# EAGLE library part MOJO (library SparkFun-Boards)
Mojo v3 FPGA Development Board Mechanical footprint with connectors for Mojo FPGA dev board. SparkFun Products: Mojo v3
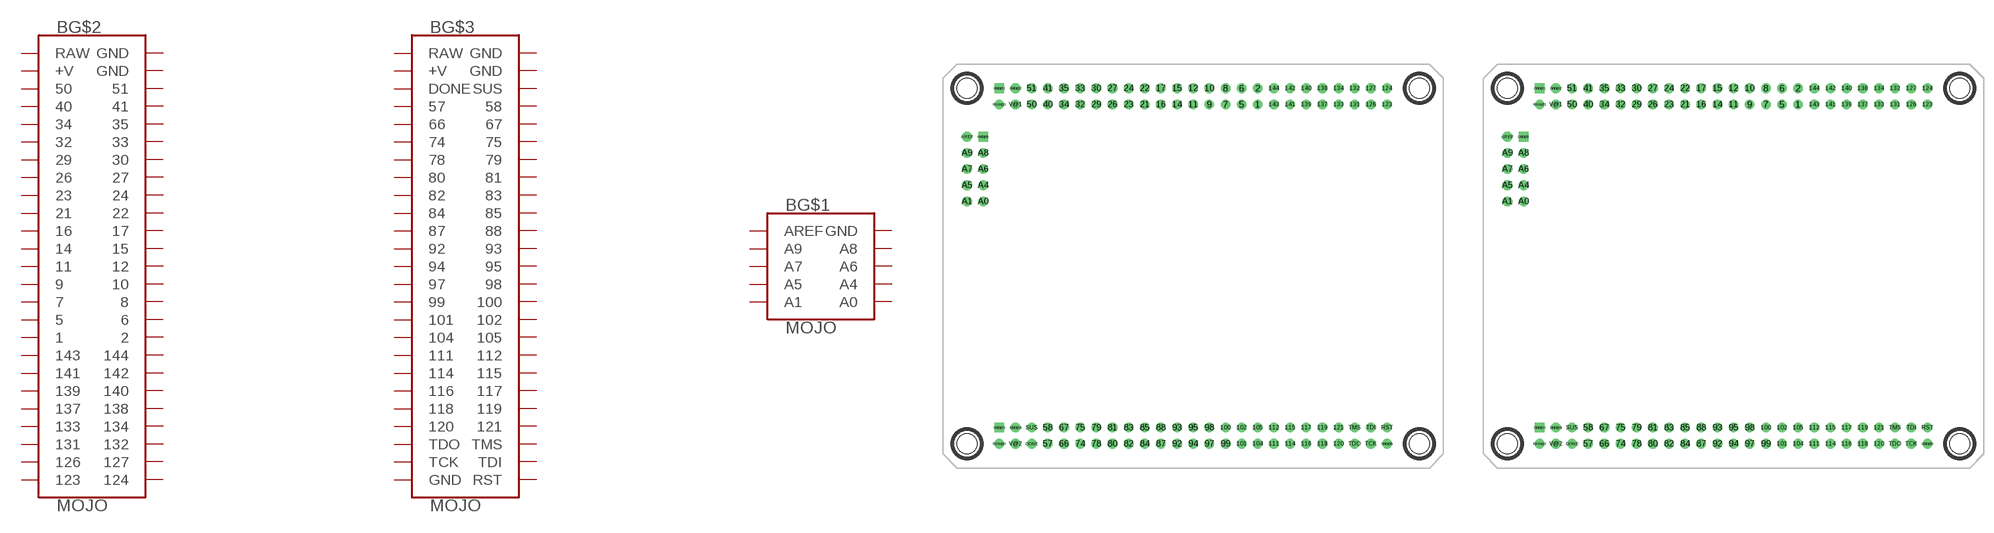
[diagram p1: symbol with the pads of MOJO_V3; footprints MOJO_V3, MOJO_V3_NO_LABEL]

Designator prefix B; gates G$1=MOJO_ANALOG_HEADER G$2=MOJO_HEADER_1 G$3=MOJO_HEADER_2

## MOJOV3  [MOJO_V3]
1  G$2:1
2  G$2:2
5  G$2:5
6  G$2:6
7  G$2:7
8  G$2:8
9  G$2:9
10  G$2:10
11  G$2:11
12  G$2:12
14  G$2:14
15  G$2:15
16  G$2:16
17  G$2:17
21  G$2:21
22  G$2:22
23  G$2:23
24  G$2:24
26  G$2:26
27  G$2:27
29  G$2:29
30  G$2:30
32  G$2:32
33  G$2:33
34  G$2:34
35  G$2:35
40  G$2:40
41  G$2:41
50  G$2:50
51  G$2:51
57  G$3:57
58  G$3:58
66  G$3:66
67  G$3:67
74  G$3:74
75  G$3:75
78  G$3:78
79  G$3:79
80  G$3:80
81  G$3:81
82  G$3:82
83  G$3:83
84  G$3:84
85  G$3:85
87  G$3:87
88  G$3:88
92  G$3:92
93  G$3:93
94  G$3:94
95  G$3:95
97  G$3:97
98  G$3:98
99  G$3:99
100  G$3:100
101  G$3:101
102  G$3:102
104  G$3:104
105  G$3:105
111  G$3:111
112  G$3:112
114  G$3:114
115  G$3:115
116  G$3:116
117  G$3:117
118  G$3:118
119  G$3:119
120  G$3:120
121  G$3:121
123  G$2:123
124  G$2:124
126  G$2:126
127  G$2:127
131  G$2:131
132  G$2:132
133  G$2:133
134  G$2:134
137  G$2:137
138  G$2:138
139  G$2:139
140  G$2:140
141  G$2:141
142  G$2:142
143  G$2:143
144  G$2:144
A0  G$1:A0  in
A1  G$1:A1  in
A4  G$1:A4  in
A5  G$1:A5  in
A6  G$1:A6  in
A7  G$1:A7  in
A8  G$1:A8  in
A9  G$1:A9  in
AREF  G$1:AREF  in
DONE  G$3:DONE
GND@1  G$2:GND  sup
GND@2  G$2:GND  sup
GND@3  G$3:GND  sup
GND@4  G$3:GND  sup
GND@5  G$1:GND  sup
GND@6  G$3:GND  sup
RAW@1  G$2:RAW  sup
RAW@2  G$3:RAW  sup
RST  G$3:RST  in
SUS  G$3:SUS  in
TCK  G$3:TCK  in
TDI  G$3:TDI  in
TDO  G$3:TDO  out
TMS  G$3:TMS  in
V@1  G$2:+V  sup
V@2  G$3:+V  sup

## MOJOV3_NO_LABEL  [MOJO_V3_NO_LABEL]
Pads as for MOJO_V3

## Footprint MOJO_V3 (pad centres in mm)
Mojo v3 FPGA Footprint Specifications: Pin count:110 Pin pitch: 0.1" Area:3.1x2.5 inch Example device(s): Mojo
drill 1: 1 10.16,24.13; 2 10.16,26.67; 5 7.62,24.13; 6 7.62,26.67; 7 5.08,24.13; 8 5.08,26.67; 9 2.54,24.13; 10 2.54,26.67; 11 0,24.13; 12 0,26.67; 14 -2.54,24.13; 15 -2.54,26.67; 16 -5.08,24.13; 17 -5.08,26.67; 21 -7.62,24.13; 22 -7.62,26.67; 23 -10.16,24.13; 24 -10.16,26.67; 26 -12.7,24.13; 27 -12.7,26.67; 29 -15.24,24.13; 30 -15.24,26.67; 32 -17.78,24.13; 33 -17.78,26.67; 34 -20.32,24.13; 35 -20.32,26.67; 40 -22.86,24.13; 41 -22.86,26.67; 50 -25.4,24.13; 51 -25.4,26.67; 57 -22.86,-29.21; 58 -22.86,-26.67; 66 -20.32,-29.21; 67 -20.32,-26.67; 74 -17.78,-29.21; 75 -17.78,-26.67; 78 -15.24,-29.21; 79 -15.24,-26.67; 80 -12.7,-29.21; 81 -12.7,-26.67; 82 -10.16,-29.21; 83 -10.16,-26.67; 84 -7.62,-29.21; 85 -7.62,-26.67; 87 -5.08,-29.21; 88 -5.08,-26.67; 92 -2.54,-29.21; 93 -2.54,-26.67; 94 0,-29.21; 95 0,-26.67; 97 2.54,-29.21; 98 2.54,-26.67; 99 5.08,-29.21; 100 5.08,-26.67; 101 7.62,-29.21; 102 7.62,-26.67; 104 10.16,-29.21; 105 10.16,-26.67; 111 12.7,-29.21; 112 12.7,-26.67; 114 15.24,-29.21; 115 15.24,-26.67; 116 17.78,-29.21; 117 17.78,-26.67; 118 20.32,-29.21; 119 20.32,-26.67; 120 22.86,-29.21; 121 22.86,-26.67; 123 30.48,24.13; 124 30.48,26.67; 126 27.94,24.13; 127 27.94,26.67; 131 25.4,24.13; 132 25.4,26.67; 133 22.86,24.13; 134 22.86,26.67; 137 20.32,24.13; 138 20.32,26.67; 139 17.78,24.13; 140 17.78,26.67; 141 15.24,24.13; 142 15.24,26.67; 143 12.7,24.13; 144 12.7,26.67; A0 -33.02,8.89; A1 -35.56,8.89; A4 -33.02,11.43; A5 -35.56,11.43; A6 -33.02,13.97; A7 -35.56,13.97; A8 -33.02,16.51; A9 -35.56,16.51; AREF -35.56,19.05; DONE -25.4,-29.21; GND@2 -27.94,26.67; GND@4 -27.94,-26.67; GND@6 30.48,-29.21; RAW@1 -30.48,24.13; RAW@2 -30.48,-29.21; RST 30.48,-26.67; SUS -25.4,-26.67; TCK 27.94,-29.21; TDI 27.94,-26.67; TDO 25.4,-29.21; TMS 25.4,-26.67; V@1 -27.94,24.13; V@2 -27.94,-29.21
drill 1 square: GND@1 -30.48,26.67; GND@3 -30.48,-26.67; GND@5 -33.02,19.05
hole 3.2 at -35.56,-29.21
hole 3.2 at -35.56,26.67
hole 3.2 at 35.56,26.67
hole 3.2 at 35.56,-29.21

## Footprint MOJO_V3_NO_LABEL (pad centres in mm)
Mojo v3 FPGA Footprint No silk labels on pins Specifications: Pin count:110 Pin pitch: 0.1" Area:3.1x2.5 inch Example device(s): Mojo
drill 1: 1 11.43,26.67; 2 11.43,29.21; 5 8.89,26.67; 6 8.89,29.21; 7 6.35,26.67; 8 6.35,29.21; 9 3.81,26.67; 10 3.81,29.21; 11 1.27,26.67; 12 1.27,29.21; 14 -1.27,26.67; 15 -1.27,29.21; 16 -3.81,26.67; 17 -3.81,29.21; 21 -6.35,26.67; 22 -6.35,29.21; 23 -8.89,26.67; 24 -8.89,29.21; 26 -11.43,26.67; 27 -11.43,29.21; 29 -13.97,26.67; 30 -13.97,29.21; 32 -16.51,26.67; 33 -16.51,29.21; 34 -19.05,26.67; 35 -19.05,29.21; 40 -21.59,26.67; 41 -21.59,29.21; 50 -24.13,26.67; 51 -24.13,29.21; 57 -21.59,-26.67; 58 -21.59,-24.13; 66 -19.05,-26.67; 67 -19.05,-24.13; 74 -16.51,-26.67; 75 -16.51,-24.13; 78 -13.97,-26.67; 79 -13.97,-24.13; 80 -11.43,-26.67; 81 -11.43,-24.13; 82 -8.89,-26.67; 83 -8.89,-24.13; 84 -6.35,-26.67; 85 -6.35,-24.13; 87 -3.81,-26.67; 88 -3.81,-24.13; 92 -1.27,-26.67; 93 -1.27,-24.13; 94 1.27,-26.67; 95 1.27,-24.13; 97 3.81,-26.67; 98 3.81,-24.13; 99 6.35,-26.67; 100 6.35,-24.13; 101 8.89,-26.67; 102 8.89,-24.13; 104 11.43,-26.67; 105 11.43,-24.13; 111 13.97,-26.67; 112 13.97,-24.13; 114 16.51,-26.67; 115 16.51,-24.13; 116 19.05,-26.67; 117 19.05,-24.13; 118 21.59,-26.67; 119 21.59,-24.13; 120 24.13,-26.67; 121 24.13,-24.13; 123 31.75,26.67; 124 31.75,29.21; 126 29.21,26.67; 127 29.21,29.21; 131 26.67,26.67; 132 26.67,29.21; 133 24.13,26.67; 134 24.13,29.21; 137 21.59,26.67; 138 21.59,29.21; 139 19.05,26.67; 140 19.05,29.21; 141 16.51,26.67; 142 16.51,29.21; 143 13.97,26.67; 144 13.97,29.21; A0 -31.75,11.43; A1 -34.29,11.43; A4 -31.75,13.97; A5 -34.29,13.97; A6 -31.75,16.51; A7 -34.29,16.51; A8 -31.75,19.05; A9 -34.29,19.05; AREF -34.29,21.59; DONE -24.13,-26.67; GND@2 -26.67,29.21; GND@4 -26.67,-24.13; GND@6 31.75,-26.67; RAW@1 -29.21,26.67; RAW@2 -29.21,-26.67; RST 31.75,-24.13; SUS -24.13,-24.13; TCK 29.21,-26.67; TDI 29.21,-24.13; TDO 26.67,-26.67; TMS 26.67,-24.13; V@1 -26.67,26.67; V@2 -26.67,-26.67
drill 1 square: GND@1 -29.21,29.21; GND@3 -29.21,-24.13; GND@5 -31.75,21.59
hole 3.2 at -34.29,-26.67
hole 3.2 at -34.29,29.21
hole 3.2 at 36.83,29.21
hole 3.2 at 36.83,-26.67

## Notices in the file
Licensing: Creative Commons ShareAlike 4.0 International - https://creativecommons.org/licenses/by-sa/4.0
